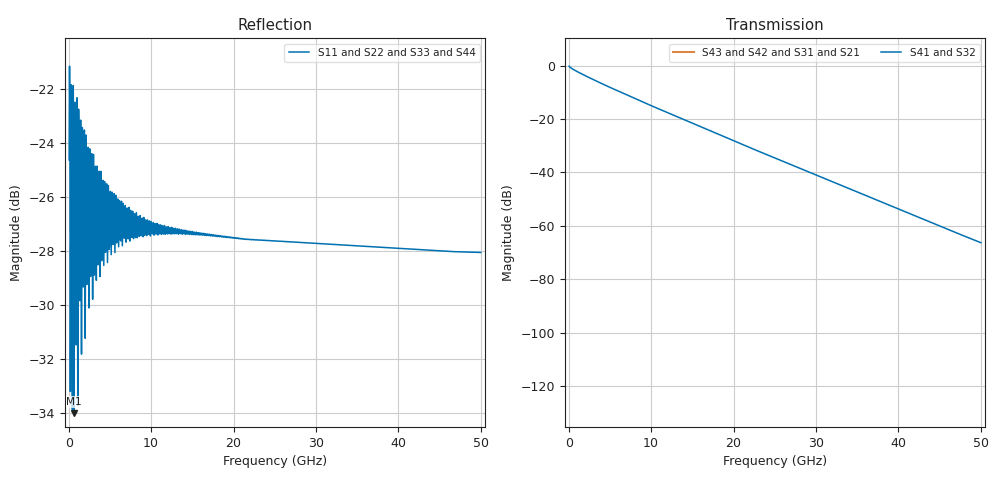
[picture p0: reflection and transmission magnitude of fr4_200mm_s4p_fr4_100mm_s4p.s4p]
! Touchstone generated by fitter/viewer
# HZ S  RI R 5.000000e+01
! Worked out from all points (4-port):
!   999 points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, 50.05 MHz to 50 GHz, reference 50 ohm
!   strongest paths, dB at 50.05 MHz, 12.51 GHz, 25.03 GHz, 37.54 GHz, 50 GHz:
!     S41: -0.2, -18.3, -34.6, -50.6, -66.3
!     S32: -0.2, -18.3, -34.6, -50.6, -66.3
!     S43: -, -, -, -, -
!     S42: -, -, -, -, -
!     S31: -, -, -, -, -
!     S21: -, -, -, -, -
!   lowest |S11| = -34.0 dB at 650.7 MHz (marker M1), VSWR 1.04, Z = 48.2 + j0.736 ohm
!   |S11| at or under -10 dB: start of sweep to end of sweep
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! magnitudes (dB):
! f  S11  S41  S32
! 50.05 MHz  -24.6  -0.2  -0.2
! 150.2 MHz  -23.2  -0.6  -0.6
! 250.3 MHz  -28.0  -0.8  -0.8
! 650.7 MHz  -34.0  -1.6  -1.6
! 9.81 GHz  -26.9  -14.8  -14.8
! 21.42 GHz  -27.5  -30.0  -30.0
! 50 GHz  -28.0  -66.3  -66.3
